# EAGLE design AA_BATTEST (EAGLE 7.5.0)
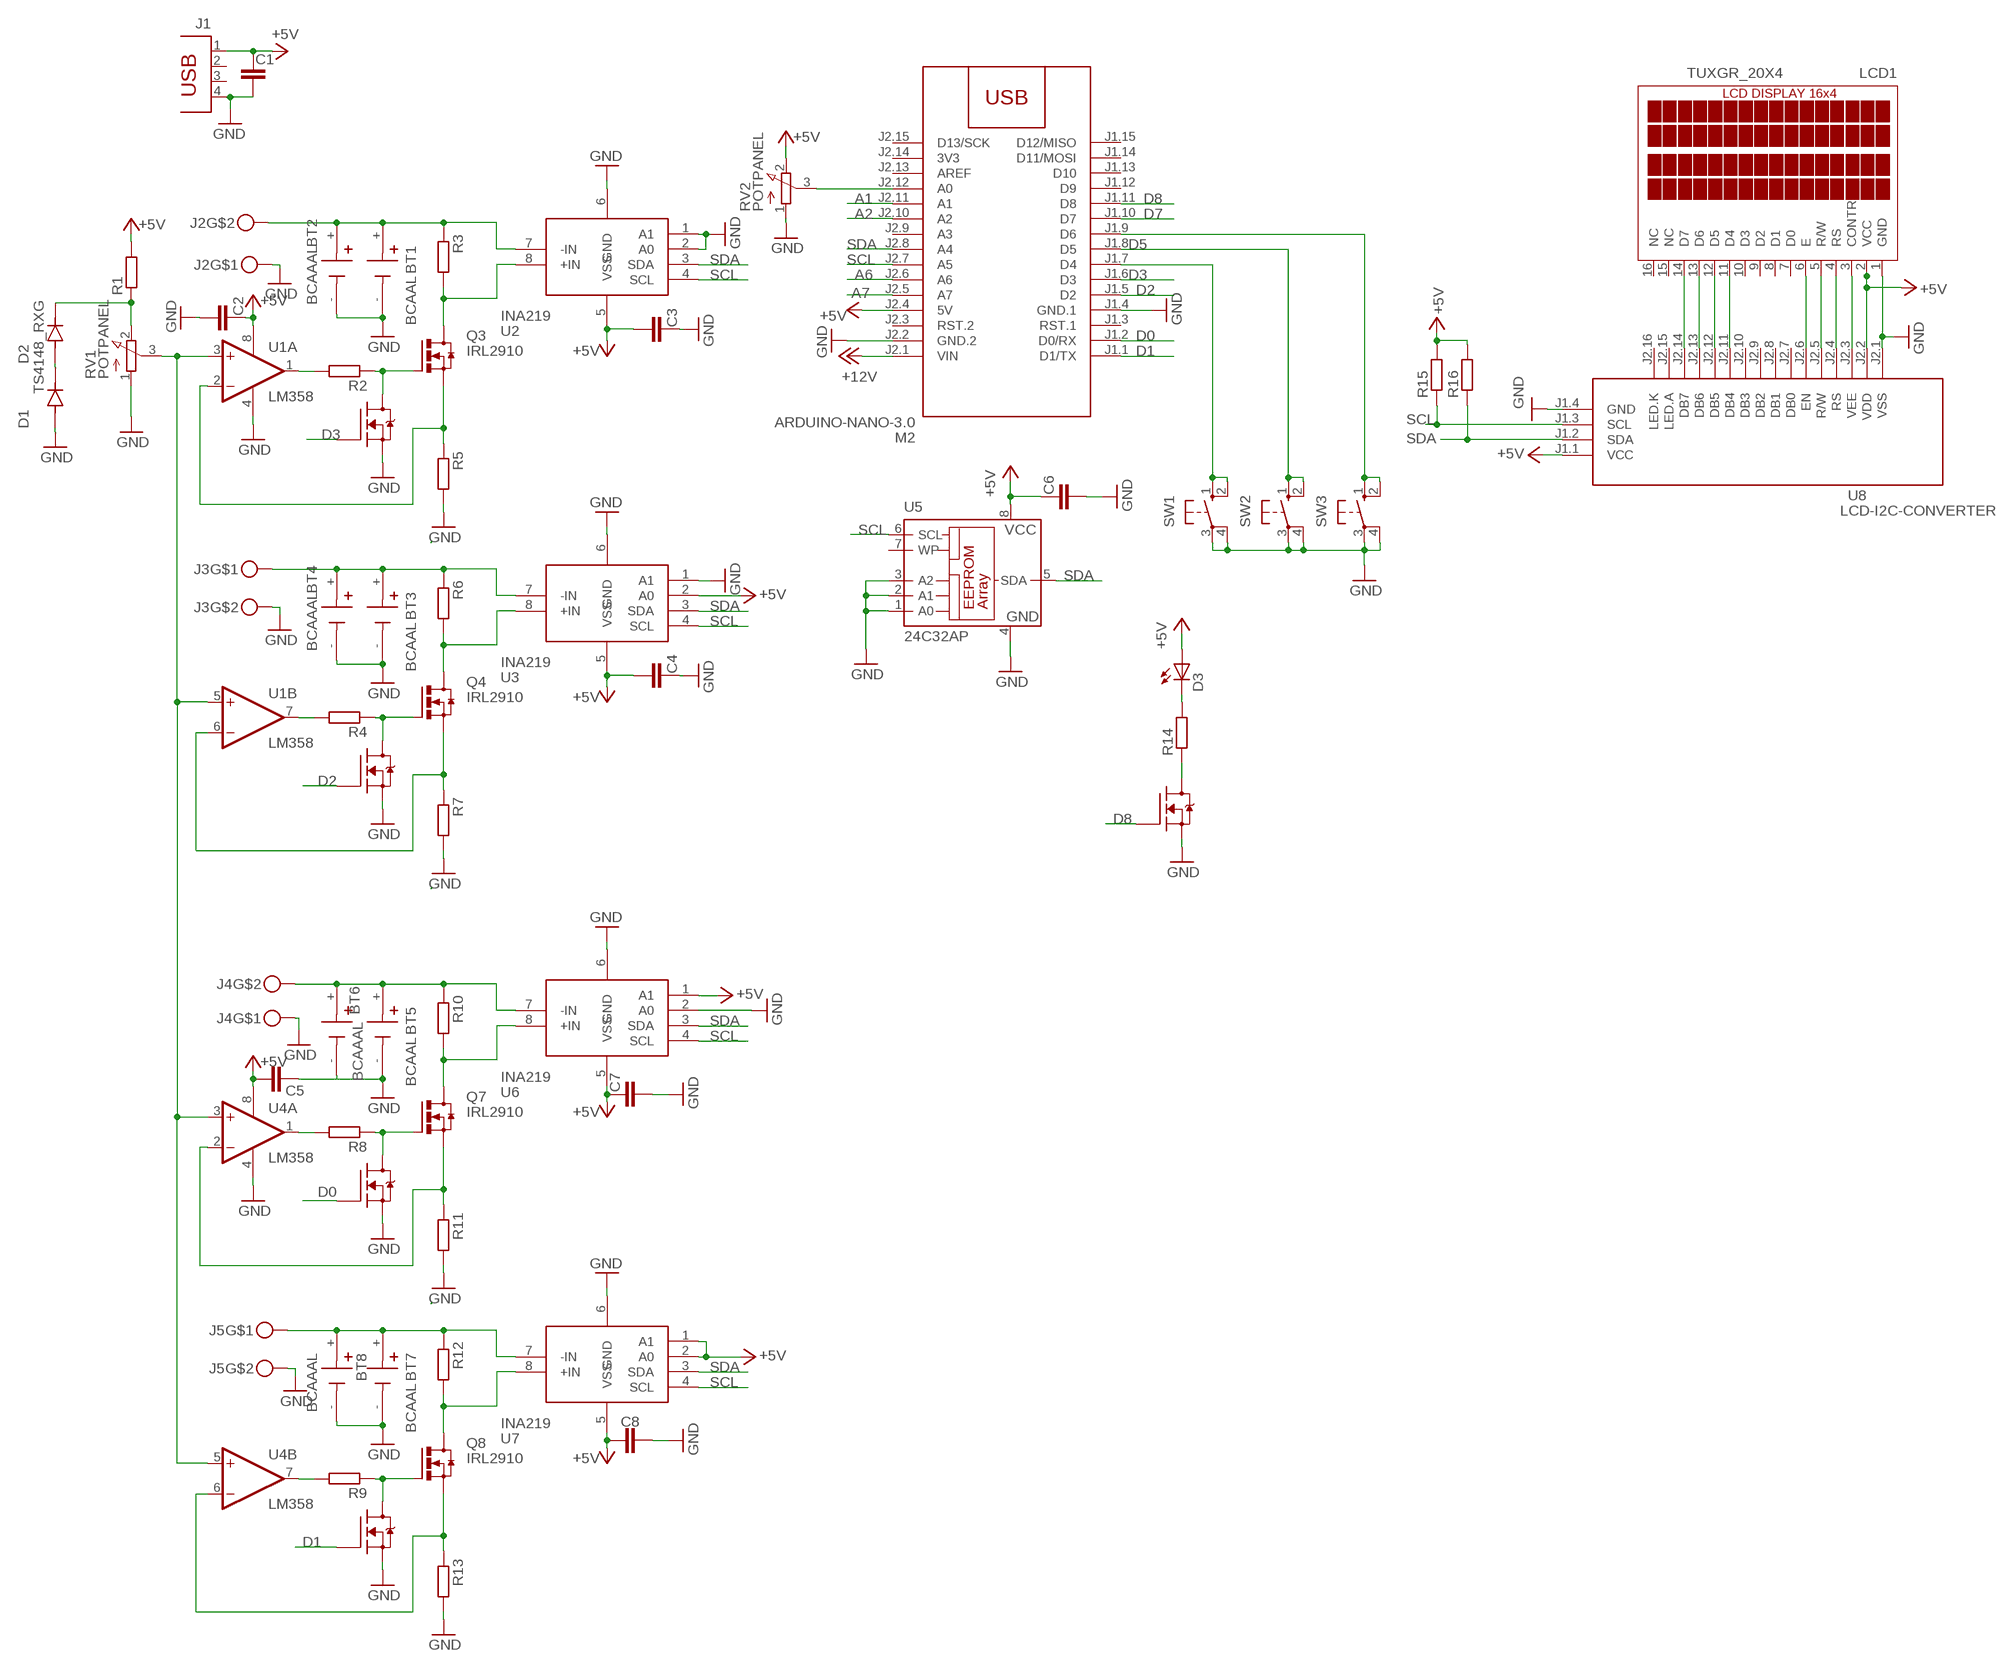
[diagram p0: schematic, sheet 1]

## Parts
BT1  BCAAL  [BAT_BCAAL]
BT2  BCAAAL  [BAT_BCAAAL]
BT3  BCAAL  [BAT_BCAAL]
BT4  BCAAAL  [BAT_BCAAAL]
BT5  BCAAL  [BAT_BCAAL]
BT6  BCAAAL  [BAT_BCAAAL]
BT7  BCAAL  [BAT_BCAAL]
BT8  BCAAAL  [BAT_BCAAAL]
C1  C-EUC1206  [C1206]
C2  C-EUC1206  [C1206]
C3  C-EUC1206  [C1206]
C4  C-EUC1206  [C1206]
C5  C-EUC1206  [C1206]
C6  C-EUC1206  [C1206]
C7  C-EUC1206  [C1206]
C8  C-EUC1206  [C1206]
D1  TS4148_RXG  [DIO_TS4148_RXG]
D2  TS4148_RXG  [DIO_TS4148_RXG]
D3  LED5MM  [LED5MM]
J1  PN87520  [PN87520]
J2  MKDSN1,5-2-5,08  [MKDSN1,5-2-5,08]
J3  MKDSN1,5-2-5,08  [MKDSN1,5-2-5,08]
J4  MKDSN1,5-2-5,08  [MKDSN1,5-2-5,08]
J5  MKDSN1,5-2-5,08  [MKDSN1,5-2-5,08]
LCD1  TUXGR_20X4  [TUXGR_20X4]
M2  ARDUINO-NANO-3.0  [ARDUINO-NANO-3.0]
Q1  ZVN3310F  [SOT23]
Q2  ZVN3310F  [SOT23]
Q3  IRL2910  [TO254P1524X483-4N]
Q4  IRL2910  [TO254P1524X483-4N]
Q5  ZVN3310F  [SOT23]
Q6  ZVN3310F  [SOT23]
Q7  IRL2910  [TO254P1524X483-4N]
Q8  IRL2910  [TO254P1524X483-4N]
Q9  ZVN3310F  [SOT23]
R1  R-EU_R1206  [R1206]
R2  R-EU_R1206  [R1206]
R3  R-EU_R2512  [R2512]
R4  R-EU_R1206  [R1206]
R5  R-EU_R2512  [R2512]
R6  R-EU_R2512  [R2512]
R7  R-EU_R2512  [R2512]
R8  R-EU_R1206  [R1206]
R9  R-EU_R1206  [R1206]
R10  R-EU_R2512  [R2512]
R11  R-EU_R2512  [R2512]
R12  R-EU_R2512  [R2512]
R13  R-EU_R2512  [R2512]
R14  R-EU_R1206  [R1206]
R15  R-EU_R1206  [R1206]
R16  R-EU_R1206  [R1206]
RV1  POTPANEL  [POTPANELP231]
RV2  POTPANEL  [POTPANELP231]
SW1  40-XX  [B3F-40XX]
SW2  40-XX  [B3F-40XX]
SW3  40-XX  [B3F-40XX]
U1  LM358  OPA2134PA  [DIL08]
U2  INA219  [SO08]
U3  INA219  [SO08]
U4  LM358  OPA2134PA  [DIL08]
U5  24C32AP  [DIL8]
U6  INA219  [SO08]
U7  INA219  [SO08]
U8  LCD-I2C-CONVERTER  [LCD-I2C-CONVERTER]

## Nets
+5V: C1.1 C2.1 C3.2 C4.2 C5.2 C6.1 C7.1 C8.1 D3.A J1.1 LCD1.2(VCC) M2.J2.4(5V) R1.2 R15.2 R16.2 RV2.2(E) U1.8(A:V+) U2.5(VSS) U3.2(A0) U3.5(VSS) U4.8(A:V+) U5.8(VCC) U6.1(A1) U6.5(VSS) U7.1(A1) U7.2(A0) U7.5(VSS) U8.J1.1(VCC) U8.J2.2(VDD)
+12V: M2.J2.1(VIN)
A1: M2.J2.11(A1)
A2: M2.J2.10(A2)
A6: M2.J2.6(A6)
A7: M2.J2.5(A7)
D0: M2.J1.2(D0/RX) Q5.2(G)
D1: M2.J1.1(D1/TX) Q6.2(G)
D2: M2.J1.5(D2) Q2.2(G)
D3: M2.J1.6(D3) Q1.2(G)
D5: M2.J1.8(D5) SW2.1(S) SW2.2(S1)
D7: M2.J1.10(D7)
D8: M2.J1.11(D8) Q9.2(G)
GND: BT1.- BT2.- BT3.- BT4.- BT5.- BT6.- BT7.- BT8.- C1.2 C2.2 C3.1 C4.1 C5.1 C6.2 C7.2 C8.2 D1.A J1.4 J2.1 J3.2 J4.1 J5.2 LCD1.1(GND) M2.J1.4(GND.1) M2.J2.2(GND.2) Q1.3(S) Q2.3(S) Q5.3(S) Q6.3(S) Q9.3(S) R5.2 R7.2 R11.2 R13.2 RV1.1(A) RV2.1(A) SW1.3(P) SW1.4(P1) SW2.3(P) SW2.4(P1) SW3.3(P) SW3.4(P1) U1.4(A:V-) U2.1(A1) U2.2(A0) U2.6(GND) U3.1(A1) U3.6(GND) U4.4(A:V-) U5.1(A0) U5.2(A1) U5.3(A2) U5.4(GND) U6.2(A0) U6.6(GND) U7.6(GND) U8.J1.4(GND) U8.J2.1(VSS)
N$1: LCD1.14(D7) U8.J2.14(DB7)
N$2: LCD1.13(D6) U8.J2.13(DB6)
N$3: LCD1.12(D5) U8.J2.12(DB5)
N$4: LCD1.11(D4) U8.J2.11(DB4)
N$5: LCD1.6(E) U8.J2.6(EN)
N$6: LCD1.5(R/W) U8.J2.5(R/W)
N$7: LCD1.4(RS) U8.J2.4(RS)
N$8: M2.J1.7(D4) SW1.1(S) SW1.2(S1)
N$9: M2.J1.9(D6) SW3.1(S) SW3.2(S1)
N$10: LCD1.3(CONTR) U8.J2.3(VEE)
N$11: D2.C(K) R1.1 RV1.2(E)
N$12: D1.C(K) D2.A
N$13: RV1.3(S) U1.3(A:+IN) U1.5(B:+IN) U4.3(A:+IN) U4.5(B:+IN)
N$14: D3.K(C) R14.2
N$15: R2.2 U1.1(A:OUT)
N$16: Q1.1(D) Q3.1(G) R2.1
N$17: Q3.4(D) R3.2 U2.8(+IN)
N$19: Q3.3(S) R5.1 U1.2(A:-IN)
N$20: R4.2 U1.7(B:OUT)
N$21: BT1.+ BT2.+ J2.2 R3.1 U2.7(-IN)
N$23: Q2.1(D) Q4.1(G) R4.1
N$25: Q4.3(S) R7.1 U1.6(B:-IN)
N$26: Q4.4(D) R6.2 U3.8(+IN)
N$27: BT3.+ BT4.+ J3.1 R6.1 U3.7(-IN)
N$28: Q9.1(D) R14.1
N$29: R8.2 U4.1(A:OUT)
N$30: Q5.1(D) Q7.1(G) R8.1
N$32: Q7.3(S) R11.1 U4.2(A:-IN)
N$33: Q7.4(D) R10.2 U6.8(+IN)
N$34: BT5.+ BT6.+ J4.2 R10.1 U6.7(-IN)
N$35: Q6.1(D) Q8.1(G) R9.1
N$36: Q8.3(S) R13.1 U4.6(B:-IN)
N$37: Q8.4(D) R12.2 U7.8(+IN)
N$38: BT7.+ BT8.+ J5.1 R12.1 U7.7(-IN)
N$39: R9.2 U4.7(B:OUT)
N$41: M2.J2.12(A0) RV2.3(S)
SCL: M2.J2.7(A5) R15.1 U2.4(SCL) U3.4(SCL) U5.6(SCL) U6.4(SCL) U7.4(SCL) U8.J1.3(SCL)
SDA: M2.J2.8(A4) R16.1 U2.3(SDA) U3.3(SDA) U5.5(SDA) U6.3(SDA) U7.3(SDA) U8.J1.2(SDA)
Unconnected: J1.2 J1.3 LCD1.7(D0) LCD1.8(D1) LCD1.9(D2) LCD1.10(D3) LCD1.15(NC) LCD1.16(NC) M2.J1.3(RST.1) M2.J1.12(D9) M2.J1.13(D10) M2.J1.14(D11/MOSI) M2.J1.15(D12/MISO) M2.J2.3(RST.2) M2.J2.9(A3) M2.J2.13(AREF) M2.J2.15(D13/SCK) U5.7(WP) U8.J2.7(DB0) U8.J2.8(DB1) U8.J2.9(DB2) U8.J2.10(DB3) U8.J2.15(LED.A) U8.J2.16(LED.K)

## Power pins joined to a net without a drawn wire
3V3: M2.J2.14(3V3)

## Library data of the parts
BT1 BT3 BT5 BT7 = BCAAL:BCAAL: AA Battery Holder Check availability; AVAILABILITY: In Stock; CHECK_PRICES: https://www.snapeda.com/parts/BCAAL/Memory+Protection+Devices/view-part/?ref=eda; DESCRIPTION: Battery Holder (Open) AA 1 Cell Solder Lug; MF: MPD (Memory Protection Devices); MP: BCAAL; PACKAGE: None; PRICE: None; SNAPEDA_LINK: https://www.snapeda.com/parts/BCAAL/Memory+Protection+Devices/view-part/?ref=snap
BT2 BT4 BT6 BT8 = BCAAAL:BCAAAL: AAA Battery Holder Check availability; AVAILABILITY: Not in stock; CHECK_PRICES: https://www.snapeda.com/parts/BCAAAL/Memory+Protection+Devices/view-part/?ref=eda; DESCRIPTION: Battery Holder (Open) AAA 1 Cell Solder Lug; MF: Memory Protection Dev.; MP: BCAAAL; PACKAGE: None; PRICE: None; SNAPEDA_LINK: https://www.snapeda.com/parts/BCAAAL/Memory+Protection+Devices/view-part/?ref=snap
C1-C8 = rcl:C-EU: CAPACITOR, European symbol
D1 D2 = TS4148_RXG:TS4148_RXG: Check availability Check availability Check availability; AVAILABILITY: In Stock; CHECK_PRICES: https://www.snapeda.com/parts/TS4148%20RXG/Taiwan+Semiconductor/view-part/?ref=eda; DESCRIPTION: 1206 (Ceramics) 75V 0.15A Switching Diode & Array; MF: Taiwan Semiconductor; MP: TS4148 RXG; PACKAGE: 1206-2 Taiwan Semiconductor; PRICE: None; SNAPEDA_LINK: https://www.snapeda.com/parts/TS4148%20RXG/Taiwan+Semiconductor/view-part/?ref=snap
D3 = led:LED: LED
J1 = con-berg:PN87520: BERG USB connector; OC_FARNELL: unknown; OC_NEWARK: unknown
J2-J5 = con-phoenix-508:MKDSN1,5-2-5,08
LCD1 = display-lcd:TUXGR_20X4: LCD DISPLAY 20X4
M2 = diy-modules:ARDUINO-NANO-3.0: Arduino Nano 3.0 and compatible devices More details available here: https://www.arduino.cc/en/Main/ArduinoBoardNano Click here to find device on ebay.com
Q1 Q2 Q5 Q6 Q9 = transistor-fet:ZVN3310F
Q3 Q4 Q7 Q8 = IRL2910STRLPBF:IRL2910
R1-R16 = rcl:R-EU_: RESISTOR, European symbol
RV1 RV2 = pot:POTPANEL
SW1-SW3 = switch-omron:40-XX: OMRON SWITCH; MF: OMRON COMPONENTS USA; MPN: B3F-4000; OC_FARNELL: 176434; OC_NEWARK: 36K3105
U1 U4 = linear:OPA2*: Dual Operational Amplifier Low Power, Single-Supply, Rail-To-Rail Operational Amplifier Source: http://focus.ti.com/lit/ds/symlink/opa2345.pdf http://focus.ti.com .. opa241.pdf http://focus.ti.com/lit/ds/symlink/opa2134.pdf
U2 U3 U6 U7 = burr-brown:INA219: Bidirectional Current/Power Monitor With I2C Interface
U5 = microchip:24*: Serial EEPROM I2C; MPN: AT24C32C-PU; OC_FARNELL: 1362652; OC_NEWARK: 50M3325
U8 = diy-modules:LCD-I2C-CONVERTER: I2C Bus to 4-Bit Parallel LCD Interface with LED backlight driver

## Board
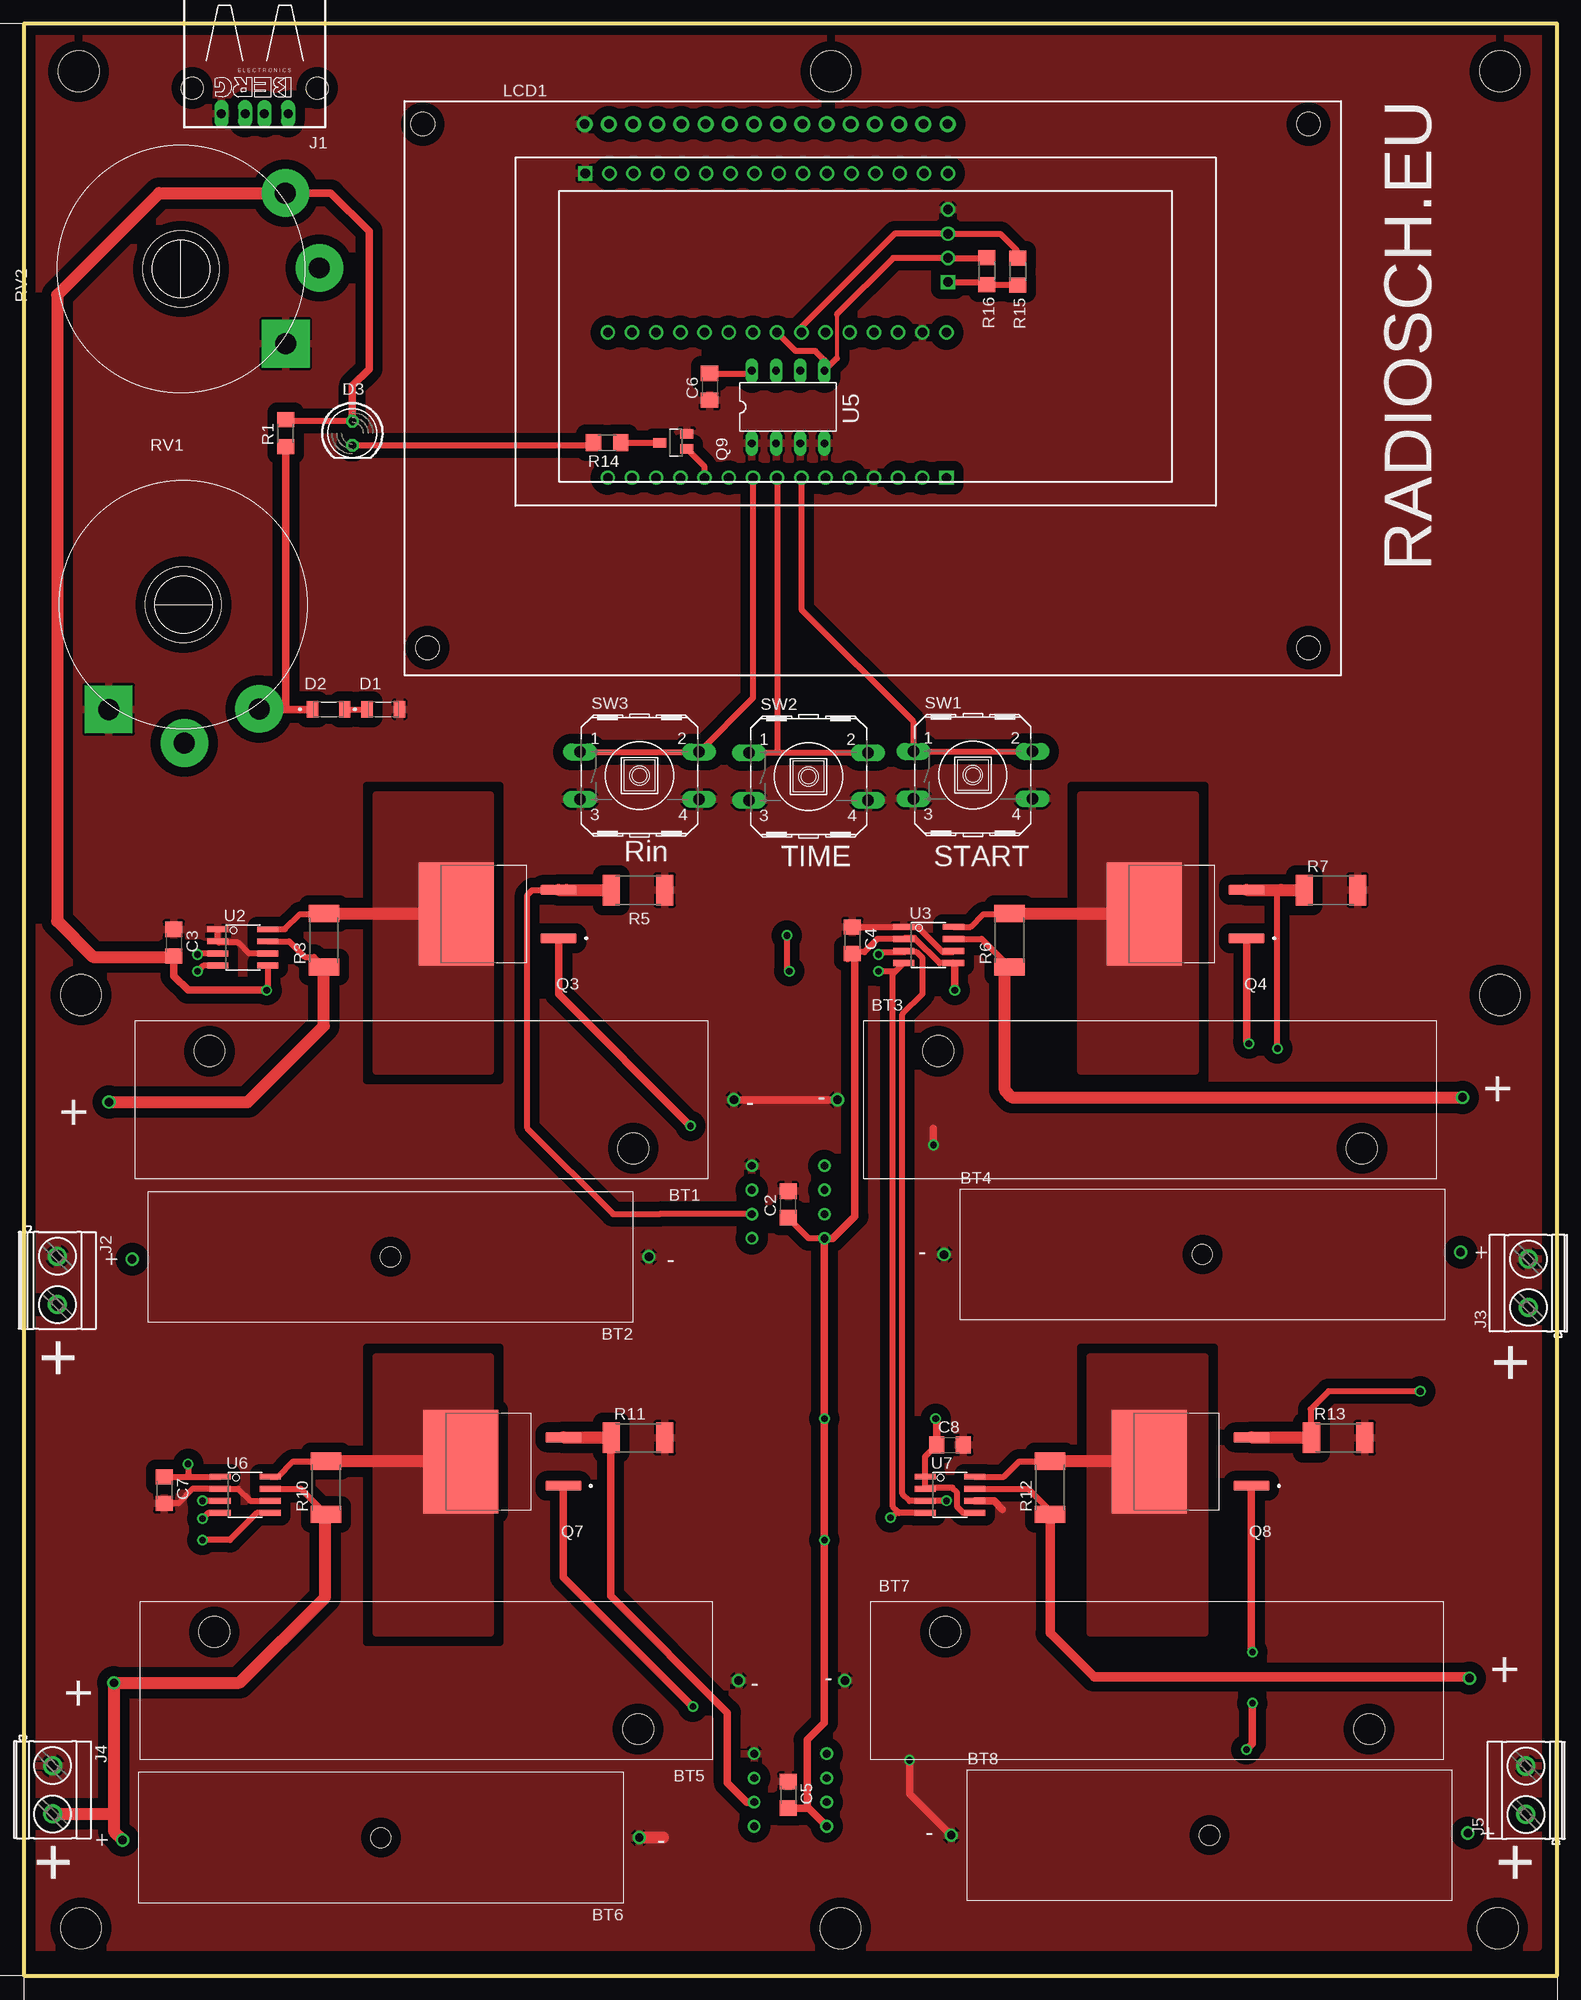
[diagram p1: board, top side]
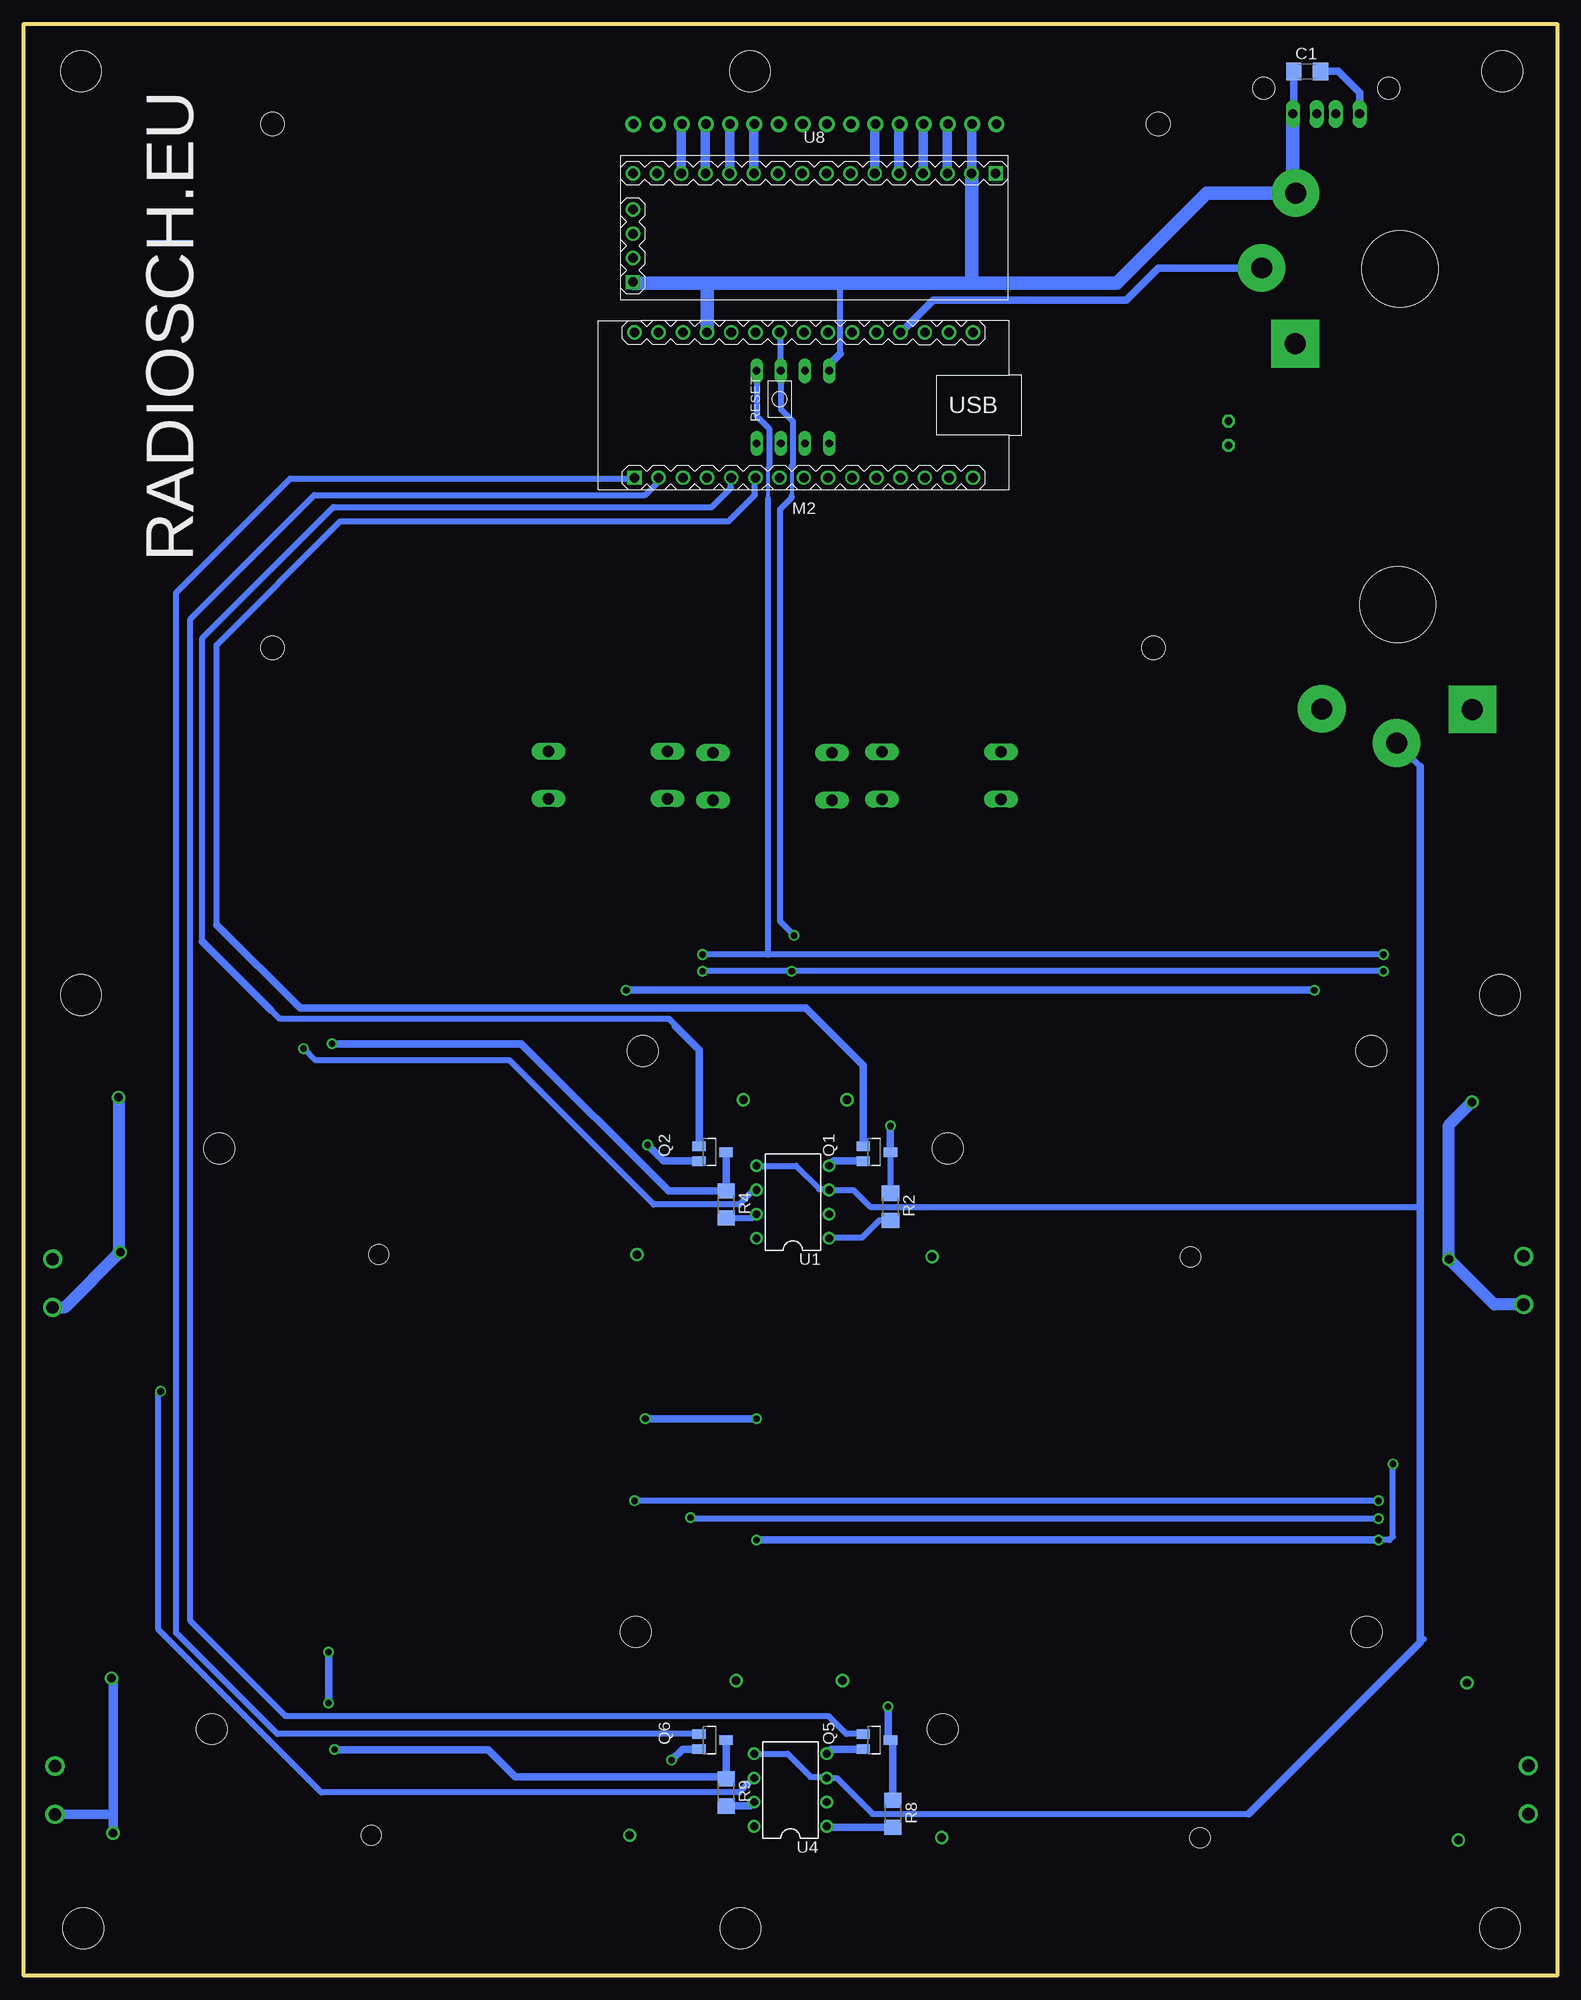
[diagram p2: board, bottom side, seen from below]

Size 161 x 205 mm. Coordinates in mm from the lower left corner, seen from the top.
Outline: 0,0 161,0 161,205 0,205 0,0
Copper layers (1*16): Top 0.035mm / dielectric 1.5mm / Bottom 0.035mm
Design rules "default *": minimum track width 10mil, minimum drill 24mil, track to track 4mil, track to pad 6mil, pad to pad 4mil, via to via 8mil, smd to smd 8mil, copper to edge 40mil, drill to drill 8mil, minimum pad ring 10mil, minimum via ring 8mil, stop-mask expansion 4mil, vias tented up to drill 0mil, thermal gap 10mil
Holes 4.3 mm at 155,103 84.75,200 155,200 5.75,200 6,103 6,5 85.75,5 154.75,5
Holes 8 mm at 16.5,179.25 16.75,144

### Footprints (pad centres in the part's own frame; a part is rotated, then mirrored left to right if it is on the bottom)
BAT_BCAAL = drill 0.89: + 32.8,0.24; - -32.8,0 | hole 3.25: 22.25,-5.1; -22.25,5.1
BAT_BCAAAL = drill 0.89: + 27.12,0.24; - -27.12,0 | hole 2.11: 0,0
C1206 = smd 1.6 x 1.8: 1 -1.4,0; 2 1.4,0
DIO_TS4148_RXG = smd 1.2 x 1.7: A 1.7,0; C -1.7,0
LED5MM = drill 0.813 octagon: A -1.27,0; K 1.27,0
PN87520 = drill 0.95 long: 1 -3.5,2.71; 2 -1,2.71; 3 1,2.71; 4 3.5,2.71 | hole 2.3: -6.57,0; 6.57,0
MKDSN1,5-2-5,08 = drill 1.3 pad 2: 1 -2.561,0.025; 2 2.519,0.025
TUXGR_20X4 = drill 1 pad 1.676: 1 11.14,-2.28; 2 13.68,-2.28; 3 16.22,-2.28; 4 18.76,-2.28; 5 21.3,-2.28; 6 23.84,-2.28; 7 26.38,-2.28; 8 28.92,-2.28; 9 31.46,-2.28; 10 34,-2.28; 11 36.54,-2.28; 12 39.08,-2.28; 13 41.62,-2.28; 14 44.16,-2.28; 15 46.7,-2.28; 16 49.24,-2.28 | hole 2.5: -5.36,-57.28; 87.14,-57.28; -5.86,-2.28; 87.14,-2.28
ARDUINO-NANO-3.0 = drill 1 square: J1.1 17.78,7.62 | drill 1: J1.2 15.24,7.62; J1.3 12.7,7.62; J1.4 10.16,7.62; J1.5 7.62,7.62; J1.6 5.08,7.62; J1.7 2.54,7.62; J1.8 0,7.62; J1.9 -2.54,7.62; J1.10 -5.08,7.62; J1.11 -7.62,7.62; J1.12 -10.16,7.62; J1.13 -12.7,7.62; J1.14 -15.24,7.62; J1.15 -17.78,7.62; J2.1 17.78,-7.62; J2.2 15.24,-7.62; J2.3 12.7,-7.62; J2.4 10.16,-7.62; J2.5 7.62,-7.62; J2.6 5.08,-7.62; J2.7 2.54,-7.62; J2.8 0,-7.62; J2.9 -2.54,-7.62; J2.10 -5.08,-7.62; J2.11 -7.62,-7.62; J2.12 -10.16,-7.62; J2.13 -12.7,-7.62; J2.14 -15.24,-7.62; J2.15 -17.78,-7.62
SOT23 = smd 1 x 1.4: 1 0,1.735; 2 -0.632,-1.1; 3 0.95,-1.1
TO254P1524X483-4N = smd 3.78 x 1.06: 1 -6.4,2.54; 3 -6.4,-2.54 | smd 7.88 x 10.84: 4 4.35,0
R1206 = smd 1.6 x 1.803: 1 -1.422,0; 2 1.422,0
R2512 = smd 1.8 x 3.2: 1 -2.8,0; 2 2.8,0
POTPANELP231 = drill 2.2 pad 5 square: 1 -7.85,-11 | drill 2.2 pad 5: 2 7.97,-10.96; 3 0.11,-14.54
B3F-40XX = drill 1.194 long: 1 -6.248,2.489; 2 6.248,2.489; 3 -6.248,-2.489; 4 6.248,-2.489
DIL08 = drill 0.813 pad 1.27: 1 -3.81,-3.81; 2 -1.27,-3.81; 3 1.27,-3.81; 4 3.81,-3.81; 5 3.81,3.81; 6 1.27,3.81; 7 -1.27,3.81; 8 -3.81,3.81
SO08 = smd 0.61 x 2.21: 1 -1.905,-2.616; 2 -0.635,-2.616; 3 0.635,-2.616; 4 1.905,-2.616; 5 1.905,2.616; 6 0.635,2.616; 7 -0.635,2.616; 8 -1.905,2.616
DIL8 = drill 0.813 long: 1 -3.81,-3.81; 2 -1.27,-3.81; 3 1.27,-3.81; 4 3.81,-3.81; 5 3.81,3.81; 6 1.27,3.81; 7 -1.27,3.81; 8 -3.81,3.81
LCD-I2C-CONVERTER = drill 1 square: J1.1 -19.05,-5.08; J2.1 19.05,6.35 | drill 1: J1.2 -19.05,-2.54; J1.3 -19.05,0; J1.4 -19.05,2.54; J2.2 16.51,6.35; J2.3 13.97,6.35; J2.4 11.43,6.35; J2.5 8.89,6.35; J2.6 6.35,6.35; J2.7 3.81,6.35; J2.8 1.27,6.35; J2.9 -1.27,6.35; J2.10 -3.81,6.35; J2.11 -6.35,6.35; J2.12 -8.89,6.35; J2.13 -11.43,6.35; J2.14 -13.97,6.35; J2.15 -16.51,6.35; J2.16 -19.05,6.35

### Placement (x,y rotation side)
BT1  41.75,92 180 top
BT2  38.5,75.5 180 top
BT3  118.25,92 0 top
BT4  123.75,75.75 0 top
BT5  42.25,31 180 top
BT6  37.5,14.5 180 top
BT7  119,31 0 top
BT8  124.5,14.75 0 top
C1  26.25,200 0 bottom
C2  80.25,81 90 top
C3  15.75,108.5 270 top
C4  87,108.75 270 top
C5  80.25,19 270 top
C6  72,166.88 270 top
C7  14.75,51 270 top
C8  97.25,55.75 0 top
D1  37.75,133 0 top
D2  32,133 0 top
D3  34.5,162 270 top
J1  24.25,198.25 180 top
J2  3.5,73 270 top
J3  158,72.75 90 top
J4  3,19.5 270 top
J5  157.75,19.5 90 top
LCD1  47.75,196.75 0 top
M2  79.1,164.95 180 bottom
Q1  71.75,86.5 270 bottom
Q2  89,86.5 270 bottom
Q3  49.75,111.5 180 top
Q4  122,111.5 180 top
Q5  71.75,24.75 270 bottom
Q6  89,24.75 270 bottom
Q7  50.25,54 180 top
Q8  122.5,54 180 top
Q9  68.5,161 90 top
R1  27.5,162 90 top
R2  70,80.75 270 bottom
R3  31.5,108.75 90 top
R4  87.25,81 270 bottom
R5  64.5,114 0 top
R6  103.5,108.75 90 top
R7  137.25,114 0 top
R8  69.75,17 270 bottom
R9  87.25,19.25 270 bottom
R10  31.75,51.25 90 top
R11  64.5,56.5 0 top
R12  107.75,51.25 90 top
R13  138,56.5 0 top
R14  61.25,161 180 top
R15  104.38,178.97 270 top
R16  101.12,179.03 270 top
RV1  16.75,144 0 top
RV2  16.5,179.25 90 top
SW1  99.65,126.1 0 top
SW2  82.4,125.95 0 top
SW3  64.65,126.05 0 top
U1  80.25,81.25 90 bottom
U2  23,108 270 top
U3  95,108.25 270 top
U4  80.5,19.5 90 bottom
U5  80.25,164.75 0 top
U6  23.25,50.5 270 top
U7  97.25,50.5 270 top
U8  78,182.95 0 bottom

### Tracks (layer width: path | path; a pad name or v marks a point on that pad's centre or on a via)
+5V  (via drill 0.7)
  Top 0.61: U3.5 96.16,106.34 93.5,109 92.5,109 U3.2 89.64,108.88 88.25,107.5 87.15,107.5 C4.2 | C7.1 17.5,52.4 | 17.5,52.4 U6.1 | U6.5 24.47,48.59 21.62,45.75 v18.75,45.75 | v17.25,53.75 17.25,52.65 17.5,52.4 | U7.5 98.66,48.59 98,49.25 98,50.75 97.5,51.25 94.75,51.25 U7.2 U7.1 94.63,54.53 C8.1 | U1.8 82.41,77.44 C2.1 | U8.J1.1 100.86,177.87 R16.2 101.17,177.55 R15.2 | C6.1 76.16,168.28 U5.8 | D3.A 27.65,163.27 R1.2 | U2.5 25.62,103.62 v25.5,103.5 | 28,187.22 RV2.2
  Top 0.813: C3.2 15.75,105 17.25,103.5 v25.5,103.5 | v97.75,103.5 97.75,106.21 U3.5 | 82.25,17.75 82.25,24.75 84.06,26.56 v84.06,45.75 v84.06,58.5 U1.8 84.94,77.44 87.25,79.75 87.25,107.1 C4.2 86.5,106.85 | 82.25,17.75 U4.8 | C5.2 82.1,17.6 82.25,17.75 | C8.1 95.85,58.4 v95.75,58.5 | D3.A 34.5,167 36.25,168.75 36.25,183.22 32.25,187.22 28,187.22
  Top 1.27: C3.2 15.65,107 7.25,107 3.5,110.75 3.5,176.5 14.22,187.22 RV2.2
  Bottom 0.61: v17.25,53.75 17.25,46.12 17.62,45.75 v18.75,45.75 | 75.25,170.38 75.25,177.75
  Bottom 0.813: v25.5,103.5 v97.75,103.5 | v95.75,58.5 v84.06,58.5 | v18.75,45.75 v84.06,45.75 | C1.1 27.65,195.64 J1.1 | U5.8 76.44,169.19 75.25,170.38
  Bottom 1.016: U8.J2.2 61.49,194.41 LCD1.2
  Bottom 1.422: J1.1 27.75,187.51 RV2.2 36.78,187.22 46.25,177.75 61.5,177.75 | 61.5,177.75 75.25,177.75 89,177.75 | 89,177.75 96.93,177.75 U8.J1.1 | M2.J2.4 89.26,177.49 89,177.75 | U8.J2.2 61.49,177.76 61.5,177.75
D0
  Bottom 0.61: Q5.2 74.63,25.38 76.5,27.25 133.5,27.25 143.5,37.25 143.5,142.5 130.5,155.5 95.75,155.5 94.5,156.75 94.5,157.17 M2.J1.2
D1
  Bottom 0.61: Q6.2 134.38,25.38 145,36 145,145.25 133,157.25 96.96,157.25 M2.J1.1
D2
  Bottom 0.61: 142.25,108.62 142.25,140.5 128.5,154.25 88.75,154.25 86.75,156.25 86.75,157.3 M2.J1.5 | 92.62,99.75 92.62,99.88 93.25,100.5 134.12,100.5 135.06,101.44
  Bottom 0.813: Q2.2 90.1,97.22 92.62,99.75 | 135.06,101.44 142.25,108.62
D3
  Bottom 0.61: 140.75,110.38 140.75,139.75 127.75,152.75 87,152.75 84.25,155.5 84.25,157.26 M2.J1.6
  Bottom 0.813: Q1.2 72.85,95.6 78.88,101.62 132,101.62 140.75,110.38
D5
  Top 0.61: SW2.1 79.25,128.44 | 79.25,128.44 SW2.2 | M2.J1.8 79.1,128.59 79.25,128.44
D8
  Top 0.61: M2.J1.11 71.48,158.49 Q9.2
GND  (via drill 0.7)
  Top 0.61: U2.1 U2.2 20.52,108.5 22.5,108.5 23.64,107.37 U2.6 | U3.6 97.5,107.5 96.5,107.5 93.84,110.16 U3.1 C4.1 | C7.2 14.78,49.62 16.25,49.62 17.76,51.13 U6.2 22.49,51.13 23.75,49.88 25.86,49.88 U6.6
  Top 0.813: U7.6 101.89,49.87 102.75,49 | BT3.- BT1.- | v95.5,87.25 95.5,89 | v93,22.62 93,19.13 BT8.-
  Top 1.27: 67.12,14.5 BT6.-
  Bottom 0.813: Q5.3 76.2,23.8 U4.4 | Q1.3 75.95,85.55 U1.4 | Q2.3 93.8,85.55 v95.5,87.25 | C1.2 23,200 20.75,197.75 J1.4 | Q6.3 91.83,23.8 v93,22.62
  pour Top (isolate 1.016, rank 5): 1,204 159,204 159,3 1,3
N$1
  Bottom 1.016: U8.J2.14 91.97,194.41 LCD1.14
N$2
  Bottom 1.016: U8.J2.13 89.43,194.41 LCD1.13
N$3
  Bottom 1.016: U8.J2.12 86.89,194.41 LCD1.12
N$4
  Bottom 1.016: U8.J2.11 84.35,194.41 LCD1.11
N$5
  Bottom 1.016: U8.J2.6 71.65,194.41 LCD1.6
N$6
  Bottom 1.016: U8.J2.5 69.11,194.41 LCD1.5
N$7
  Bottom 1.016: U8.J2.4 66.57,194.41 LCD1.4
N$8
  Top 0.61: M2.J1.7 81.64,143.49 93.38,131.75 93.38,128.62 SW1.1 SW1.2
N$9
  Top 0.61: M2.J1.9 76.56,134.2 SW3.2 SW3.1
N$10
  Bottom 1.016: U8.J2.3 64.03,194.41 LCD1.3
N$11
  Top 0.813: R1.1 27.5,133.25 27.25,133 | D2.C 27.25,133 | 27.25,133 24.76,133 RV1.2
N$12
  Top 0.61: D2.A D1.C
N$13
  Bottom 0.61: U1.5 79.94,85.06 77.5,82.62 76.55,82.62 U1.3 73.89,82.52 72.12,80.75 14.62,80.75 14.38,80.5 | U4.5 80.81,23.31 78.38,20.88 76.8,20.88 U4.3 75.64,20.77 71.88,17 32.38,17 | 14.38,126.97 RV1.3 | 14.38,35 14,35.38
  Bottom 0.813: 32.38,17 14.38,35 14.38,80.5 14.38,126.97
N$14
  Top 0.61: D3.K 59.56,160.73 R14.2
N$15
  Bottom 0.61: R2.2 71.17,79.33 73,77.5 76.38,77.5 U1.1
N$16  (via drill 0.7)
  Top 0.813: Q3.1 56.15,103.1 v70,89.25
  Bottom 0.61: Q1.1 70.02,82.19 R2.1
  Bottom 0.813: v70,89.25 70,86.52 Q1.1
N$17
  Top 0.61: U2.8 27.41,109.91 29,111.5 31.45,111.5 R3.2
  Top 1.27: R3.2 45.35,111.55 Q3.4
  pour Top (isolate 1.27, rank 2, no thermals): 37,124 49,124 49,95 37,95
N$19
  Top 0.61: U1.2 66.77,79.98 66.75,80 61.88,80 52.88,89 52.88,113.5 53.38,114 56.96,114 57,114.04
  Top 1.27: Q3.3 57,114.04 61.66,114.04 R5.1
N$20
  Bottom 0.61: R4.2 84.46,79.58 U1.7
N$21
  Top 0.61: U2.7 27.86,108.63 29.5,107 30.45,107 R3.1
  Top 1.27: BT1.+ 23.51,91.76 31.5,99.75 R3.1
  Bottom 1.27: BT1.+ 11.38,89.33 BT2.+ 6.6,70.48 J2.2
N$23  (via drill 0.7)
  Top 0.813: Q4.1 128.4,98.1 v128.62,97.88
  Bottom 0.813: v128.62,97.88 108.75,97.88 93.3,82.42 R4.1 87.25,86.48 Q2.1
N$25  (via drill 0.7)
  Top 0.61: v131.62,97.38 131.62,113.66 132,114.04
  Top 1.27: Q4.3 132,114.04 134.41,114.04 R7.1
  Bottom 0.61: U1.6 84.36,82.52 85.88,81 94.88,81 110,96.12 130.38,96.12 v131.62,97.38
N$26
  Top 0.61: U3.8 99.41,110.16 100.75,111.5 103.95,111.5 104,111.55
  Top 1.27: R6.2 104,111.55 117.6,111.55 Q4.4
  pour Top (isolate 1.27, rank 2, no thermals): 111,124 123,124 123,95 111,95
N$27
  Top 0.61: U3.7 100.56,108.88 R6.1
  Top 1.27: BT3.+ 103.75,92.25 103,93 103,105.45 R6.1
  Bottom 1.27: BT3.+ 151.05,76.17 BT4.+ 156.67,70.19 J3.1
N$28
  Top 0.61: R14.1 Q9.1
N$29
  Bottom 0.813: R8.2 76.58,15.58 U4.1
N$30  (via drill 0.7)
  Top 0.813: Q7.1 56.65,41.85 v70.25,28.25
  Bottom 0.813: v70.25,28.25 70.25,24.98 Q5.1 69.75,24.48 R8.1
N$32
  Top 0.813: U4.2 75.89,18.23 73.88,20.25 73.88,27.62 61.62,39.88 61.62,56.42 R11.1
  Top 1.27: Q7.3 61.66,56.54 R11.1
N$33
  Top 0.61: U6.8 26.66,52.41 28.25,54 31.7,54 R10.2
  Top 1.27: Q7.4 31.8,54 R10.2
  pour Top (isolate 1.27, rank 2, no thermals): 37,65 49,65 49,36 37,36
N$34
  Top 0.61: U6.7 29.07,51.13 R10.1
  Top 1.27: R10.1 31.62,48.33 31.62,39.75 22.64,30.76 BT5.+ 9.45,16.75 | 9.45,16.75 9.45,15.19 BT6.+ | J4.2 9.22,16.98 9.45,16.75
N$35  (via drill 0.7)
  Top 0.813: Q8.1 128.9,34.1 v129,34 | v129,28.62 129,24.38 v128.38,23.75
  Bottom 0.813: Q6.1 87.25,24.73 R9.1 87.45,20.88 109.38,20.88 112.25,23.75 v128.38,23.75 | v129,34 v129,28.62
N$36  (via drill 0.7)
  Top 0.61: v146.62,61.38 137,61.38 135.12,59.5 135.12,57.04 134.62,56.54
  Top 1.27: Q8.3 134.62,56.54 135.16,56.54 R13.1
  Bottom 0.61: U4.6 84.36,20.77 85.88,19.25 129.75,19.25 146.88,36.38 146.88,61.25 v146.62,61.38
N$37
  Top 0.61: U7.8 102.91,52.41 104.5,54 107.7,54 R12.2
  Top 1.27: Q8.4 107.8,54 R12.2
  pour Top (isolate 1.27, rank 2, no thermals): 112,65 124,65 124,36 112,36
N$38
  Top 0.61: U7.7 105.49,51.13 107.62,49 107.62,48.58 R12.1
  Top 1.016: R12.1 107.75,36 112.38,31.38 151.66,31.38 BT7.+
  Bottom 1.016: BT8.+ 151.62,16.88 | 151.62,16.88 151.62,31.06 BT7.+ | J5.1 151.68,16.94 151.62,16.88
N$39
  Bottom 0.813: R9.2 84.71,17.83 U4.7
N$41
  Bottom 0.813: RV2.3 41.89,179.36 45.25,176 65.51,176 M2.J2.12
SCL  (via drill 0.7)
  Top 0.61: U2.4 18.84,106.09 v18.25,105.5 | v89.75,105.5 91.54,105.5 | 91.54,105.5 U3.4 | v80.12,109.25 80.12,105.75 v80.38,105.5 | U7.4 91.91,48.59 91.75,48.75 | 91.75,48.75 91.25,49.25 91.25,105.21 91.54,105.5 | U6.4 19.34,48.59 v18.75,48 | v91,48.12 91.12,48.12 91.75,48.75 | M2.J2.7 81.64,173.14 91.5,183 97,183 U8.J1.3 102.55,182.95 104.25,181.25 104.25,180.52 R15.1
  Bottom 0.406: 80.38,158.5 80.38,155.38
  Bottom 0.61: v18.25,105.5 v80.38,105.5 v89.75,105.5 | 80.38,158.5 80.25,158.62 80.25,163.25 81.52,164.52 U5.6 81.52,172.45 M2.J2.7 | 80.38,155.38 80.38,155.25 81.62,154 81.62,110.75 v80.12,109.25 | v18.75,48 90.88,48 v91,48.12
SDA  (via drill 0.7)
  Top 0.406: 85.38,174.5 85.38,169.88
  Top 0.61: U2.3 18.36,107.37 v18.25,107.25 | v89.75,107.25 90,107.5 92.27,107.5 U3.3 92.5,107.5 93.75,107.5 94.38,106.88 94.38,103.12 92.25,101 92.25,50.62 93.01,49.87 U7.3 94.64,49.88 v96.88,49.88 | U6.3 18.76,49.87 v18.75,49.88 | M2.J2.8 81.05,170.62 83.12,170.62 84.06,169.69 U5.5 85.38,169.88 | 85.38,174.5 91.28,180.41 U8.J1.2 101.09,180.41 R16.1
  Bottom 0.406: 82.88,158.25 82.88,155.12
  Bottom 0.61: v18.25,107.25 82.88,107.25 | 82.88,107.25 v89.75,107.25 | U5.5 84.06,163.81 82.75,162.5 82.75,158.38 82.88,158.25 | 82.88,155.12 82.88,107.25 | v18.75,49.88 v96.88,49.88

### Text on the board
tPlace: RADIOSCH.EU | Rin | TIME | START | + | + | + | +
bPlace: RADIOSCH.EU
